(* Logix 5000 AddOnInstructionDefinition export Banner_LM_Param_v4; software revision 33.00; part 2 of 2 *)
(* tags used below, declared in another part *)
   LM : Banner_LM_v4;
   Port_Data : Banner_IOL_Port_v4;
   Port : INT;
   Local_Control : DINT;
   Command_Being_Processed : BOOL;
   Update_Archive : BOOL;
   Index_Write_Inprocess : INT;
   Index_Write_Control : INT;
   Inprocess_Index : DINT;
(* Banner_LM_Param_v4, continued *)

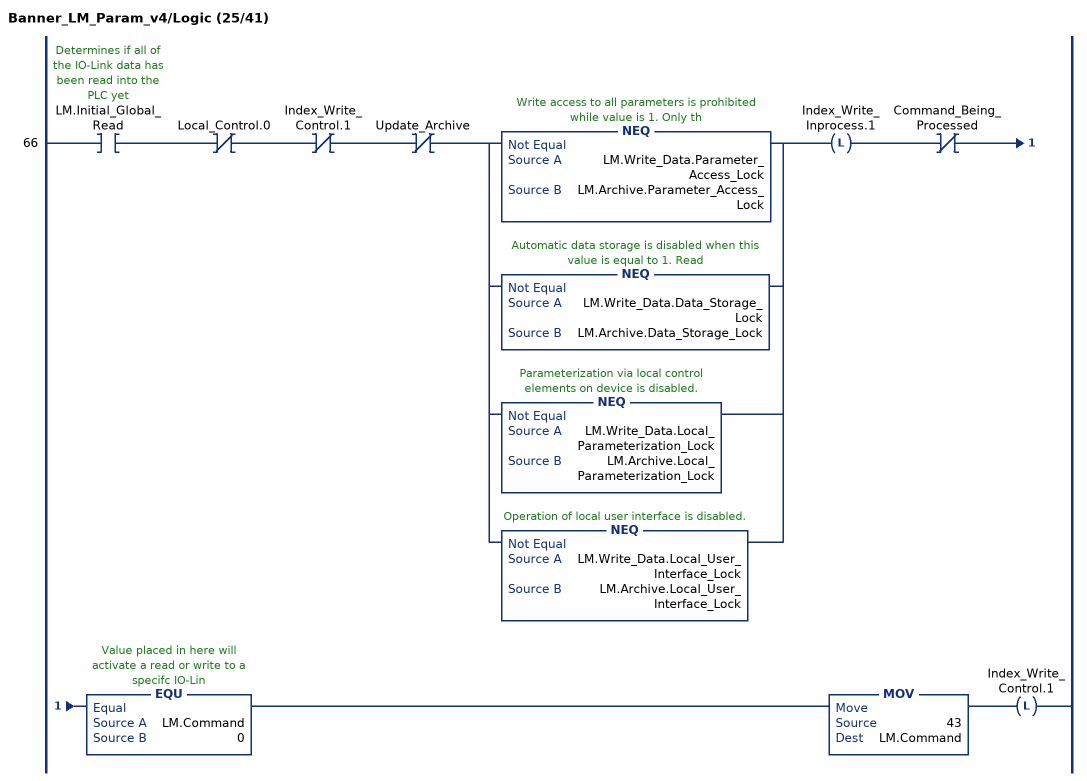
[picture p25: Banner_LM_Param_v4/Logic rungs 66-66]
   66: XIC(LM.Initial_Global_Read)XIO(Local_Control.0)XIO(Index_Write_Control.1)XIO(Update_Archive)[NEQ(LM.Write_Data.Parameter_Access_Lock,LM.Archive.Parameter_Access_Lock) ,NEQ(LM.Write_Data.Data_Storage_Lock,LM.Archive.Data_Storage_Lock) ,NEQ(LM.Write_Data.Local_Parameterization_Lock,LM.Archive.Local_Parameterization_Lock) ,NEQ(LM.Write_Data.Local_User_Interface_Lock,LM.Archive.Local_User_Interface_Lock) ]OTL(Index_Write_Inprocess.1)XIO(Command_Being_Processed)EQU(LM.Command,0)MOV(43,LM.Command)OTL(Index_Write_Control.1);
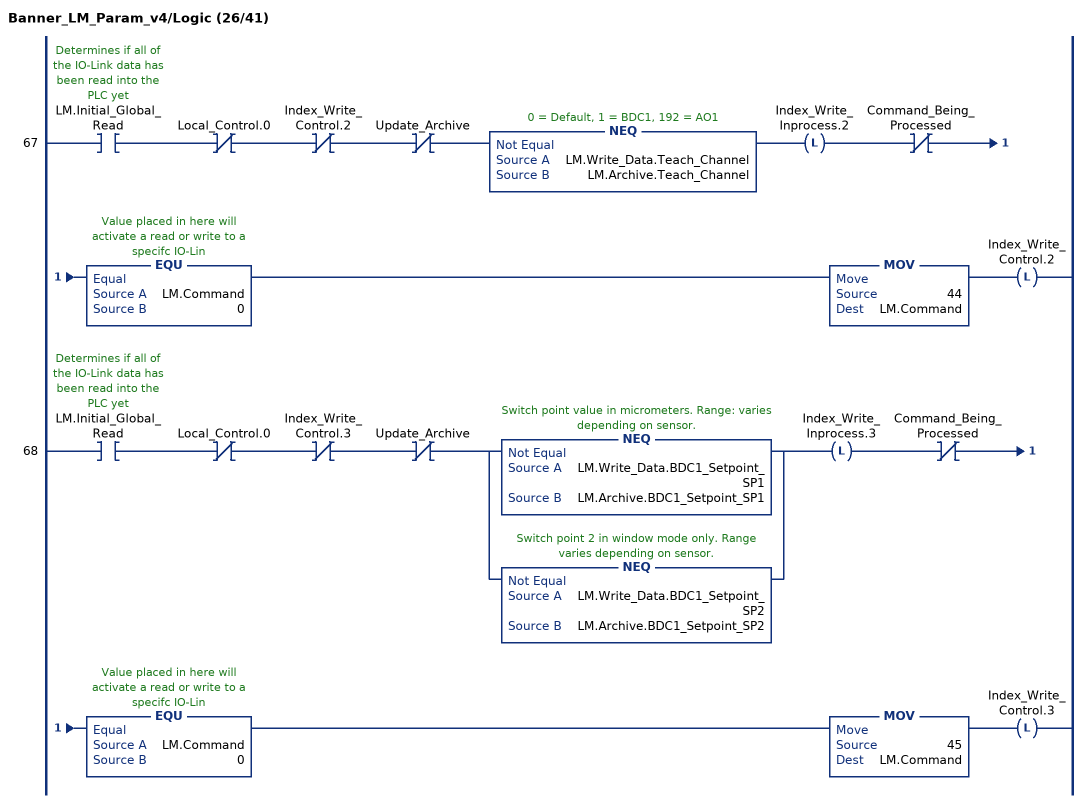
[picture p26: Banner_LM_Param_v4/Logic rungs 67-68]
   67: XIC(LM.Initial_Global_Read)XIO(Local_Control.0)XIO(Index_Write_Control.2)XIO(Update_Archive)NEQ(LM.Write_Data.Teach_Channel,LM.Archive.Teach_Channel)OTL(Index_Write_Inprocess.2)XIO(Command_Being_Processed)EQU(LM.Command,0)MOV(44,LM.Command)OTL(Index_Write_Control.2);
   68: XIC(LM.Initial_Global_Read)XIO(Local_Control.0)XIO(Index_Write_Control.3)XIO(Update_Archive)[NEQ(LM.Write_Data.BDC1_Setpoint_SP1,LM.Archive.BDC1_Setpoint_SP1) ,NEQ(LM.Write_Data.BDC1_Setpoint_SP2,LM.Archive.BDC1_Setpoint_SP2) ]OTL(Index_Write_Inprocess.3)XIO(Command_Being_Processed)EQU(LM.Command,0)MOV(45,LM.Command)OTL(Index_Write_Control.3);
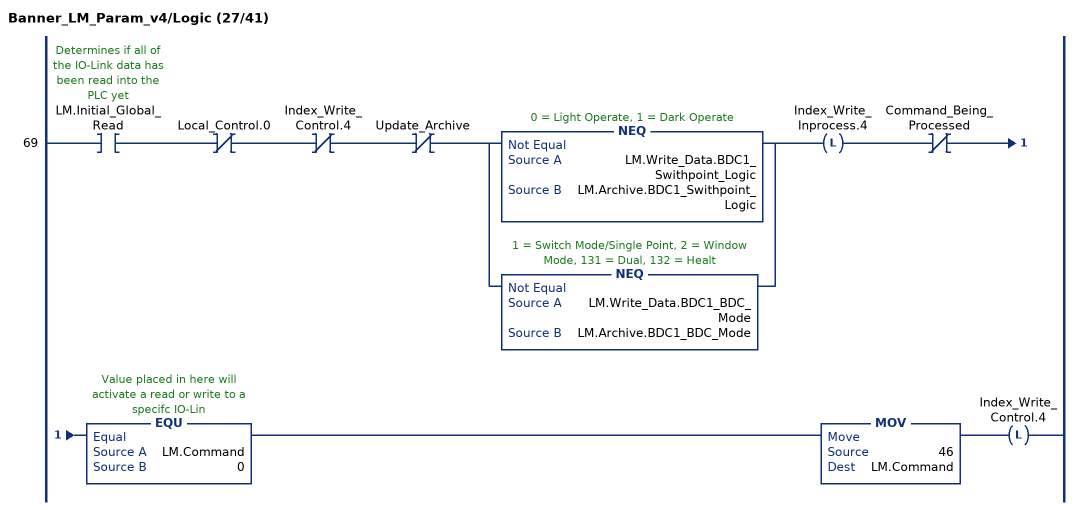
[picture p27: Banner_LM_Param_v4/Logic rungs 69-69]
   69: XIC(LM.Initial_Global_Read)XIO(Local_Control.0)XIO(Index_Write_Control.4)XIO(Update_Archive)[NEQ(LM.Write_Data.BDC1_Swithpoint_Logic,LM.Archive.BDC1_Swithpoint_Logic) ,NEQ(LM.Write_Data.BDC1_BDC_Mode,LM.Archive.BDC1_BDC_Mode) ]OTL(Index_Write_Inprocess.4)XIO(Command_Being_Processed)EQU(LM.Command,0)MOV(46,LM.Command)OTL(Index_Write_Control.4);
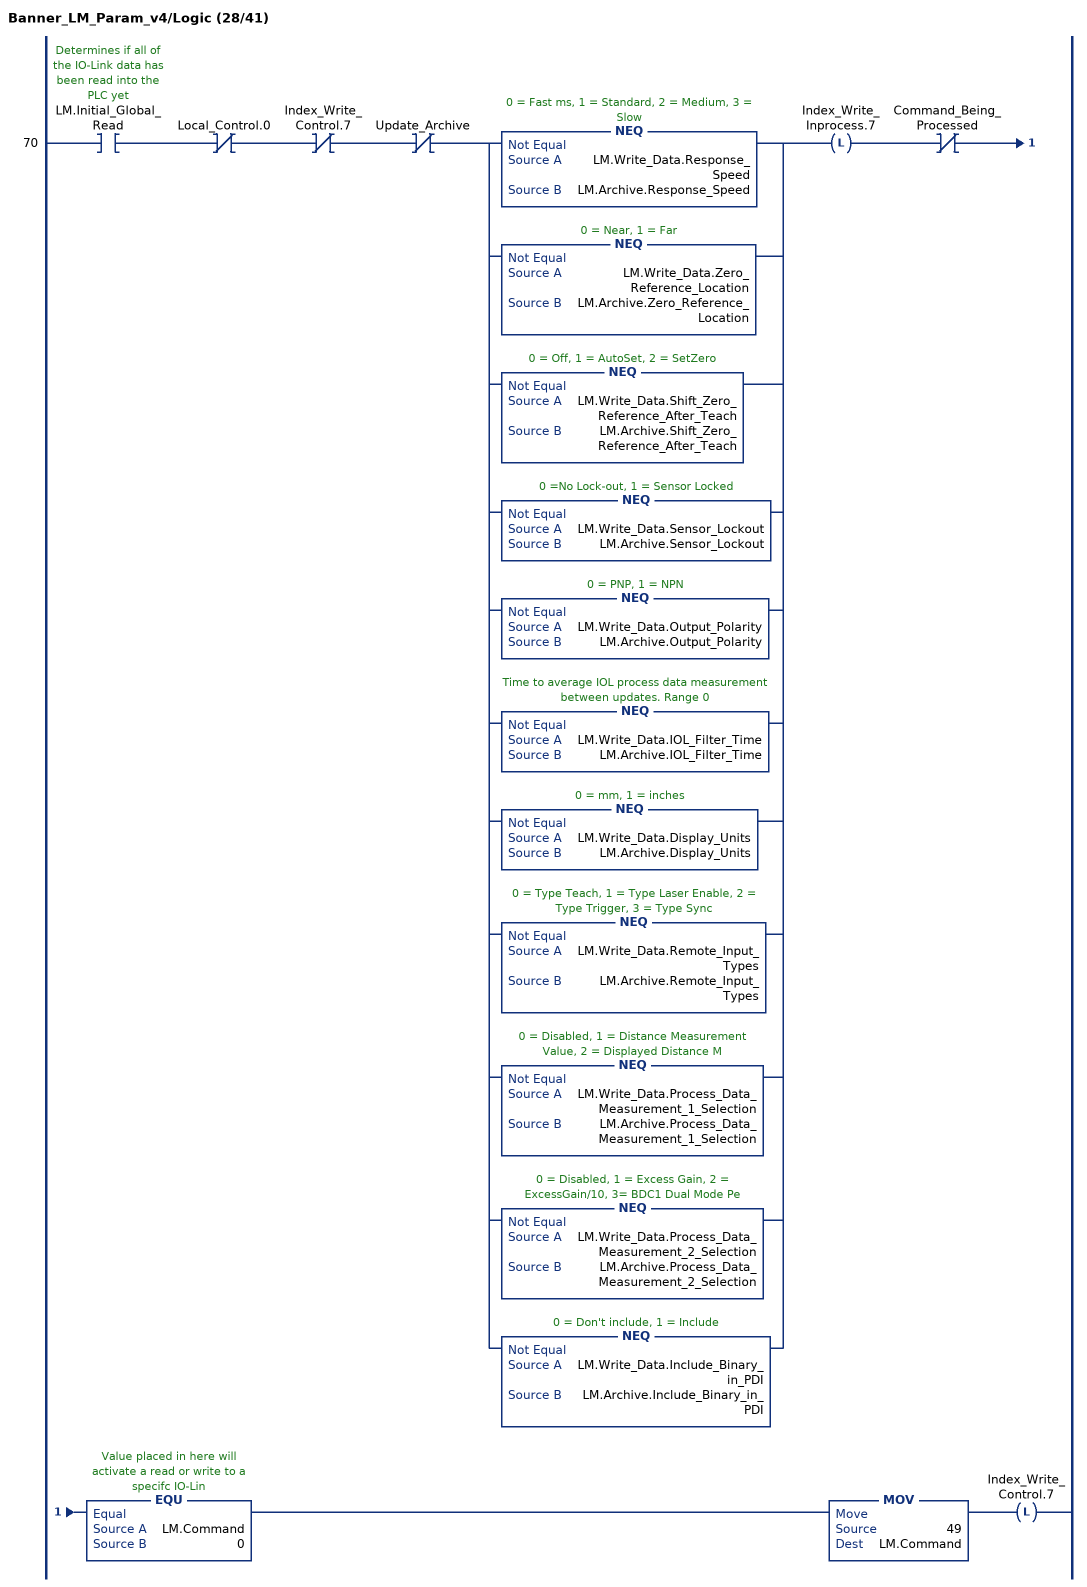
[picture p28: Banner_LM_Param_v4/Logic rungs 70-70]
   70: XIC(LM.Initial_Global_Read)XIO(Local_Control.0)XIO(Index_Write_Control.7)XIO(Update_Archive)[NEQ(LM.Write_Data.Response_Speed,LM.Archive.Response_Speed) ,NEQ(LM.Write_Data.Zero_Reference_Location,LM.Archive.Zero_Reference_Location) ,NEQ(LM.Write_Data.Shift_Zero_Reference_After_Teach,LM.Archive.Shift_Zero_Reference_After_Teach) ,NEQ(LM.Write_Data.Sensor_Lockout,LM.Archive.Sensor_Lockout) ,NEQ(LM.Write_Data.Output_Polarity,LM.Archive.Output_Polarity) ,NEQ(LM.Write_Data.IOL_Filter_Time,LM.Archive.IOL_Filter_Time) ,NEQ(LM.Write_Data.Display_Units,LM.Archive.Display_Units) ,NEQ(LM.Write_Data.Remote_Input_Types,LM.Archive.Remote_Input_Types) ,NEQ(LM.Write_Data.Process_Data_Measurement_1_Selection,LM.Archive.Process_Data_Measurement_1_Selection) ,NEQ(LM.Write_Data.Process_Data_Measurement_2_Selection,LM.Archive.Process_Data_Measurement_2_Selection) ,NEQ(LM.Write_Data.Include_Binary_in_PDI,LM.Archive.Include_Binary_in_PDI) ]OTL(Index_Write_Inprocess.7)XIO(Command_Being_Processed)EQU(LM.Command,0)MOV(49,LM.Command)OTL(Index_Write_Control.7);
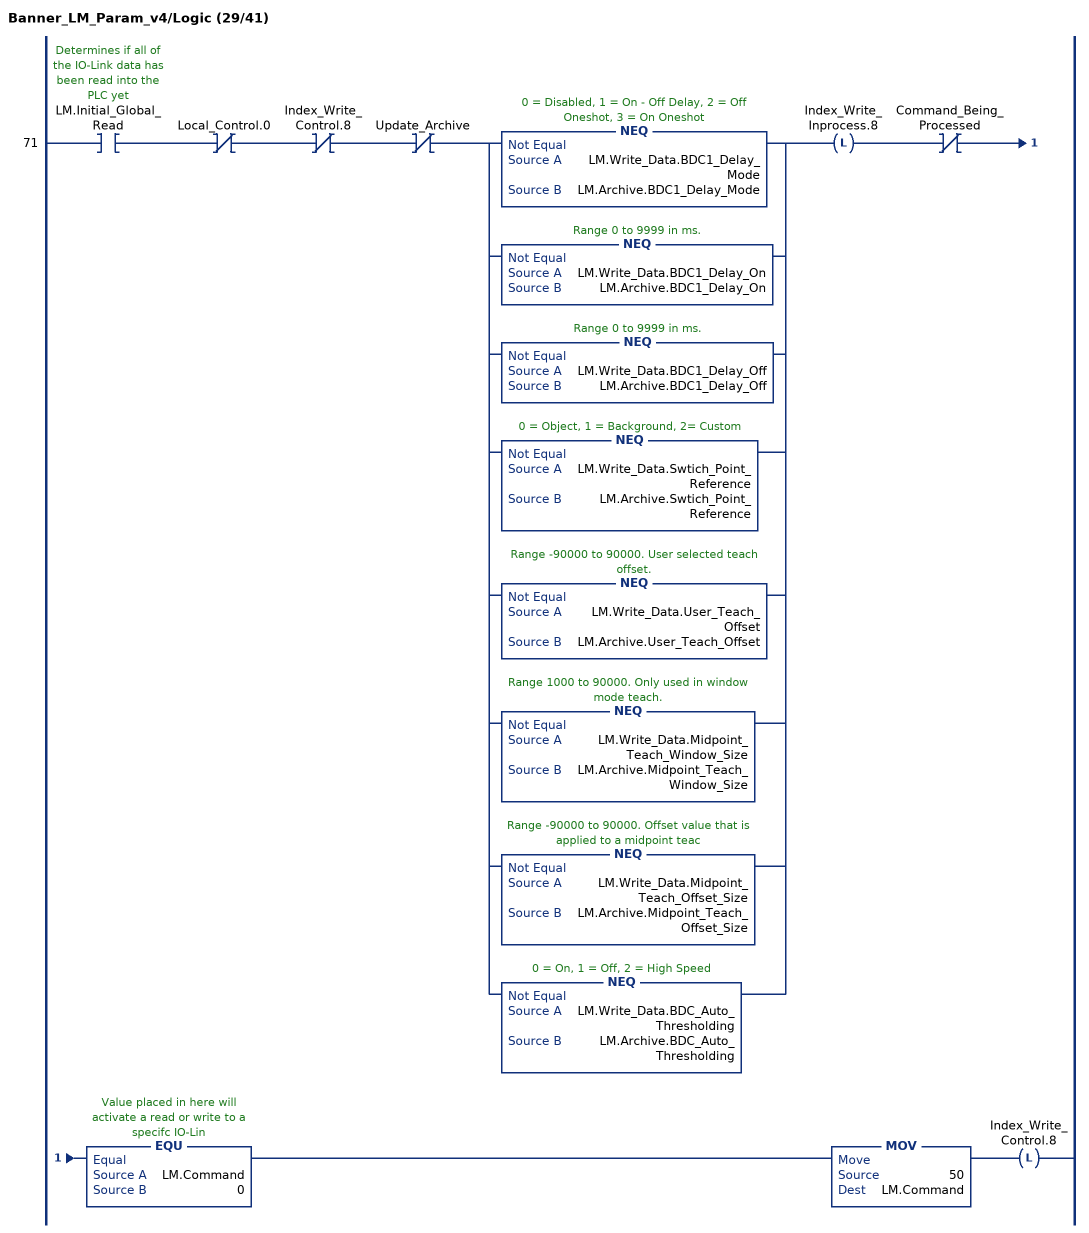
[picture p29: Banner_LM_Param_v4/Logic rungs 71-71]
   71: XIC(LM.Initial_Global_Read)XIO(Local_Control.0)XIO(Index_Write_Control.8)XIO(Update_Archive)[NEQ(LM.Write_Data.BDC1_Delay_Mode,LM.Archive.BDC1_Delay_Mode) ,NEQ(LM.Write_Data.BDC1_Delay_On,LM.Archive.BDC1_Delay_On) ,NEQ(LM.Write_Data.BDC1_Delay_Off,LM.Archive.BDC1_Delay_Off) ,NEQ(LM.Write_Data.Swtich_Point_Reference,LM.Archive.Swtich_Point_Reference) ,NEQ(LM.Write_Data.User_Teach_Offset,LM.Archive.User_Teach_Offset) ,NEQ(LM.Write_Data.Midpoint_Teach_Window_Size,LM.Archive.Midpoint_Teach_Window_Size) ,NEQ(LM.Write_Data.Midpoint_Teach_Offset_Size,LM.Archive.Midpoint_Teach_Offset_Size) ,NEQ(LM.Write_Data.BDC_Auto_Thresholding,LM.Archive.BDC_Auto_Thresholding) ]OTL(Index_Write_Inprocess.8)XIO(Command_Being_Processed)EQU(LM.Command,0)MOV(50,LM.Command)OTL(Index_Write_Control.8);
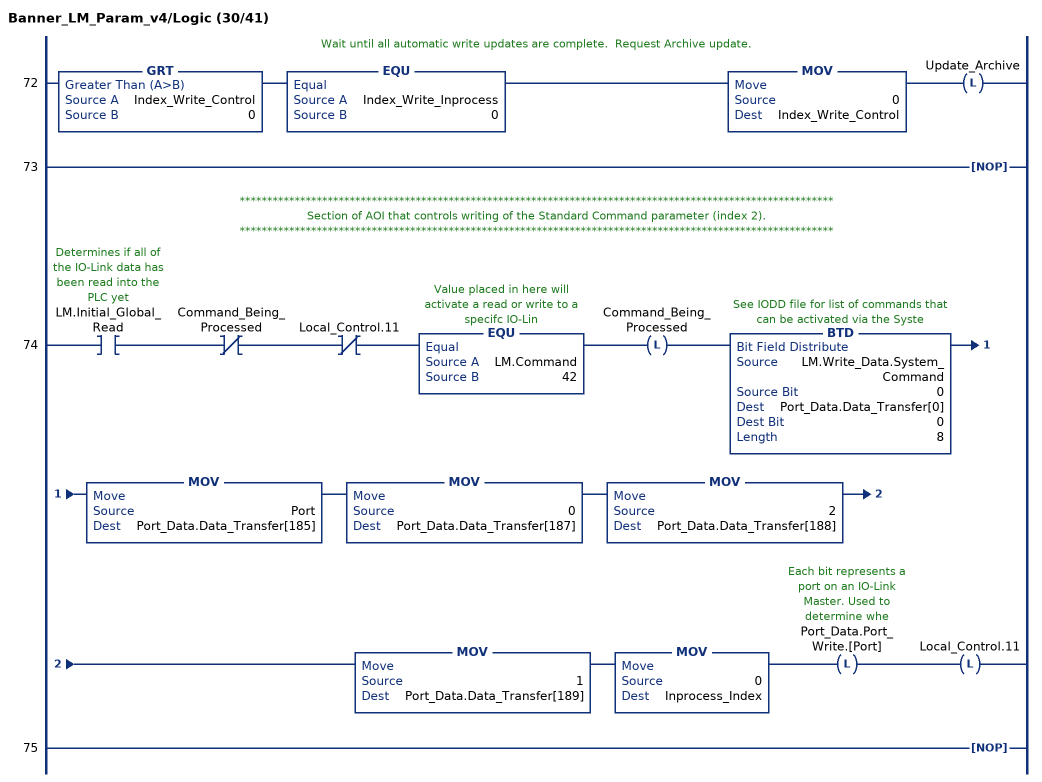
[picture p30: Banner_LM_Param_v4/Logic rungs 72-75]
   // Wait until all automatic write updates are complete.  Request Archive update.
   72: GRT(Index_Write_Control,0)EQU(Index_Write_Inprocess,0)MOV(0,Index_Write_Control)OTL(Update_Archive);
   73: NOP();
   // ************************************************************************************************************
   // Section of AOI that controls writing of the Standard Command parameter (index 2).
   // ************************************************************************************************************
   74: XIC(LM.Initial_Global_Read)XIO(Command_Being_Processed)XIO(Local_Control.11)EQU(LM.Command,42)OTL(Command_Being_Processed)BTD(LM.Write_Data.System_Command,0,Port_Data.Data_Transfer[0],0,8)MOV(Port,Port_Data.Data_Transfer[185])MOV(0,Port_Data.Data_Transfer[187])MOV(2,Port_Data.Data_Transfer[188])MOV(1,Port_Data.Data_Transfer[189])MOV(0,Inprocess_Index)OTL(Port_Data.Port_Write.[Port])OTL(Local_Control.11);
   75: NOP();
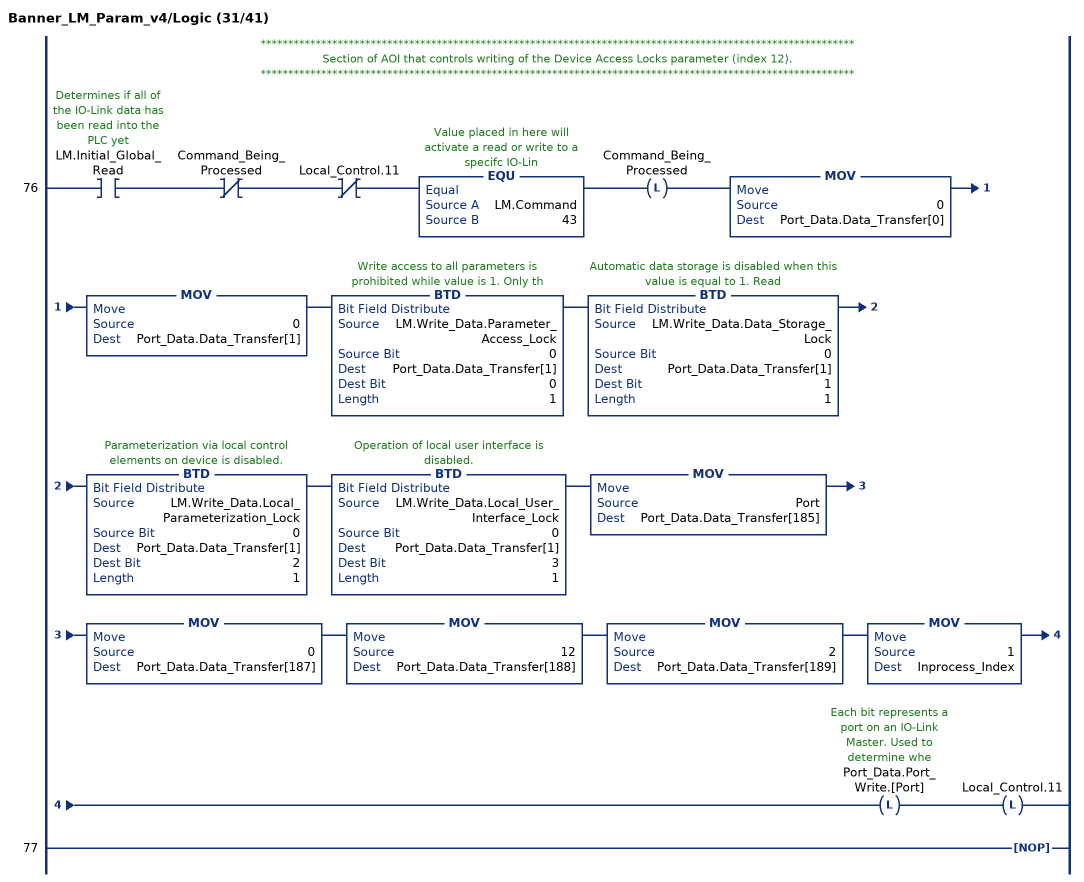
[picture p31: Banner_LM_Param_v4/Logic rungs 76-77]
   // ************************************************************************************************************
   // Section of AOI that controls writing of the Device Access Locks parameter (index 12).
   // ************************************************************************************************************
   76: XIC(LM.Initial_Global_Read)XIO(Command_Being_Processed)XIO(Local_Control.11)EQU(LM.Command,43)OTL(Command_Being_Processed)MOV(0,Port_Data.Data_Transfer[0])MOV(0,Port_Data.Data_Transfer[1])BTD(LM.Write_Data.Parameter_Access_Lock,0,Port_Data.Data_Transfer[1],0,1)BTD(LM.Write_Data.Data_Storage_Lock,0,Port_Data.Data_Transfer[1],1,1)BTD(LM.Write_Data.Local_Parameterization_Lock,0,Port_Data.Data_Transfer[1],2,1)BTD(LM.Write_Data.Local_User_Interface_Lock,0,Port_Data.Data_Transfer[1],3,1)MOV(Port,Port_Data.Data_Transfer[185])MOV(0,Port_Data.Data_Transfer[187])MOV(12,Port_Data.Data_Transfer[188])MOV(2,Port_Data.Data_Transfer[189])MOV(1,Inprocess_Index)OTL(Port_Data.Port_Write.[Port])OTL(Local_Control.11);
   77: NOP();
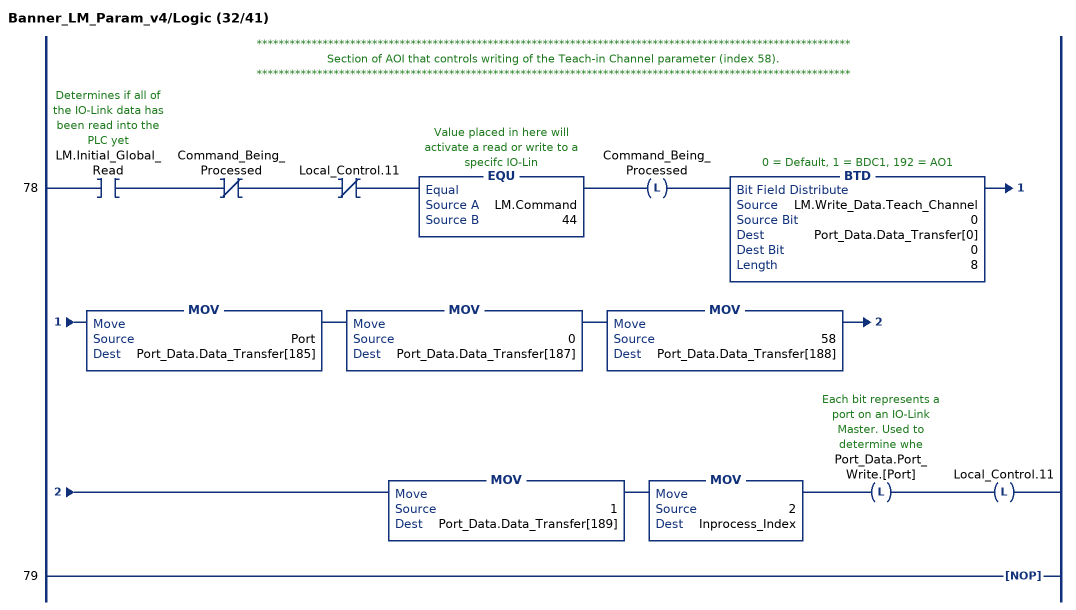
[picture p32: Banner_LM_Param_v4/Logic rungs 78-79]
   // ************************************************************************************************************
   // Section of AOI that controls writing of the Teach-in Channel parameter (index 58).
   // ************************************************************************************************************
   78: XIC(LM.Initial_Global_Read)XIO(Command_Being_Processed)XIO(Local_Control.11)EQU(LM.Command,44)OTL(Command_Being_Processed)BTD(LM.Write_Data.Teach_Channel,0,Port_Data.Data_Transfer[0],0,8)MOV(Port,Port_Data.Data_Transfer[185])MOV(0,Port_Data.Data_Transfer[187])MOV(58,Port_Data.Data_Transfer[188])MOV(1,Port_Data.Data_Transfer[189])MOV(2,Inprocess_Index)OTL(Port_Data.Port_Write.[Port])OTL(Local_Control.11);
   79: NOP();
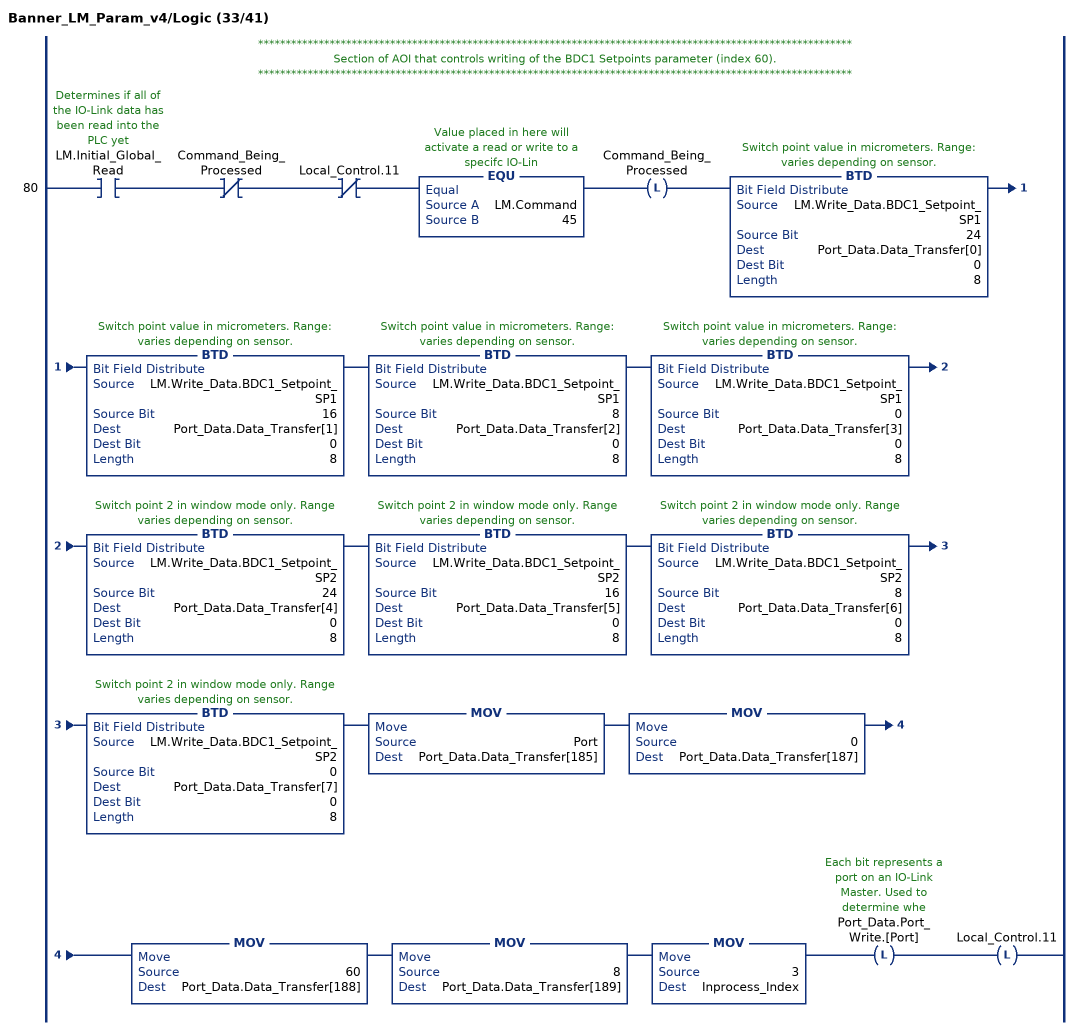
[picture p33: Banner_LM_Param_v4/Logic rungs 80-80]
   // ************************************************************************************************************
   // Section of AOI that controls writing of the BDC1 Setpoints parameter (index 60).
   // ************************************************************************************************************
   80: XIC(LM.Initial_Global_Read)XIO(Command_Being_Processed)XIO(Local_Control.11)EQU(LM.Command,45)OTL(Command_Being_Processed)BTD(LM.Write_Data.BDC1_Setpoint_SP1,24,Port_Data.Data_Transfer[0],0,8)BTD(LM.Write_Data.BDC1_Setpoint_SP1,16,Port_Data.Data_Transfer[1],0,8)BTD(LM.Write_Data.BDC1_Setpoint_SP1,8,Port_Data.Data_Transfer[2],0,8)BTD(LM.Write_Data.BDC1_Setpoint_SP1,0,Port_Data.Data_Transfer[3],0,8)BTD(LM.Write_Data.BDC1_Setpoint_SP2,24,Port_Data.Data_Transfer[4],0,8)BTD(LM.Write_Data.BDC1_Setpoint_SP2,16,Port_Data.Data_Transfer[5],0,8)BTD(LM.Write_Data.BDC1_Setpoint_SP2,8,Port_Data.Data_Transfer[6],0,8)BTD(LM.Write_Data.BDC1_Setpoint_SP2,0,Port_Data.Data_Transfer[7],0,8)MOV(Port,Port_Data.Data_Transfer[185])MOV(0,Port_Data.Data_Transfer[187])MOV(60,Port_Data.Data_Transfer[188])MOV(8,Port_Data.Data_Transfer[189])MOV(3,Inprocess_Index)OTL(Port_Data.Port_Write.[Port])OTL(Local_Control.11);
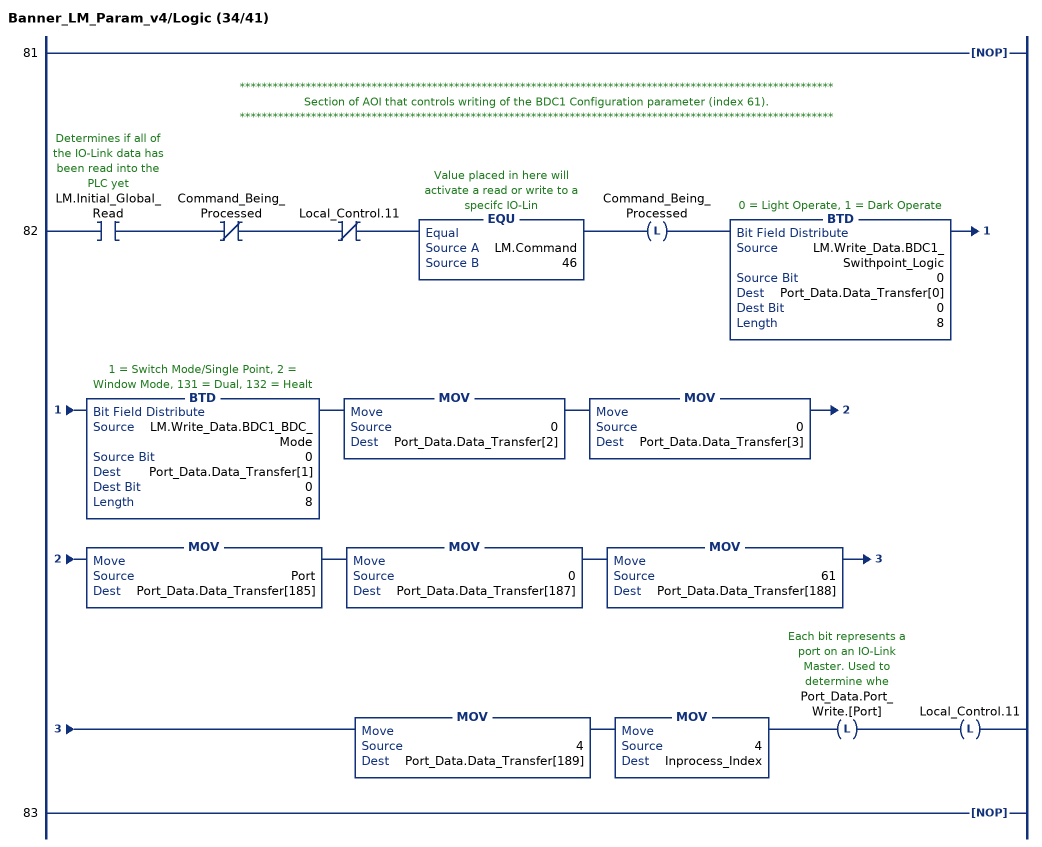
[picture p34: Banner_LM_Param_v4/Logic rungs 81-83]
   81: NOP();
   // ************************************************************************************************************
   // Section of AOI that controls writing of the BDC1 Configuration parameter (index 61).
   // ************************************************************************************************************
   82: XIC(LM.Initial_Global_Read)XIO(Command_Being_Processed)XIO(Local_Control.11)EQU(LM.Command,46)OTL(Command_Being_Processed)BTD(LM.Write_Data.BDC1_Swithpoint_Logic,0,Port_Data.Data_Transfer[0],0,8)BTD(LM.Write_Data.BDC1_BDC_Mode,0,Port_Data.Data_Transfer[1],0,8)MOV(0,Port_Data.Data_Transfer[2])MOV(0,Port_Data.Data_Transfer[3])MOV(Port,Port_Data.Data_Transfer[185])MOV(0,Port_Data.Data_Transfer[187])MOV(61,Port_Data.Data_Transfer[188])MOV(4,Port_Data.Data_Transfer[189])MOV(4,Inprocess_Index)OTL(Port_Data.Port_Write.[Port])OTL(Local_Control.11);
   83: NOP();
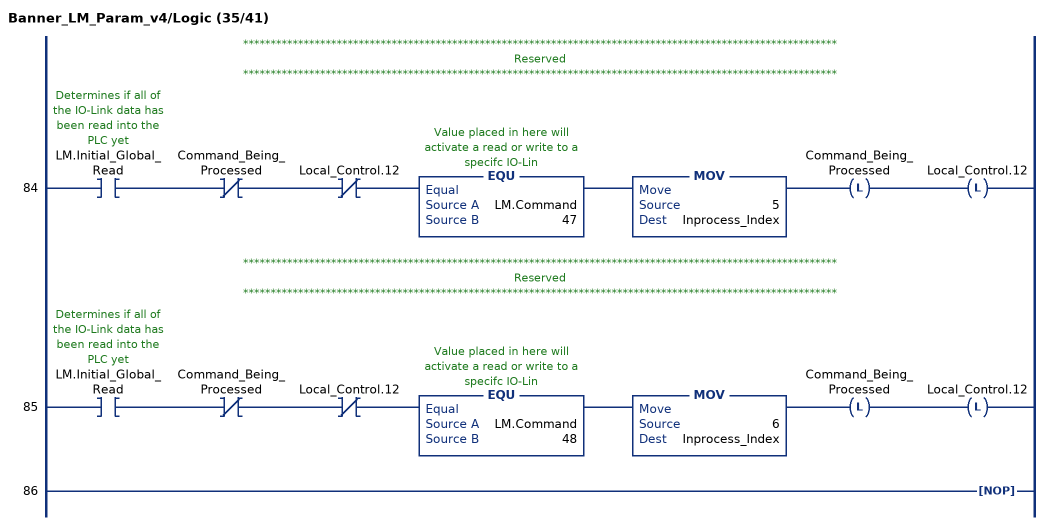
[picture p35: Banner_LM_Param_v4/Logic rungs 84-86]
   // ************************************************************************************************************
   // Reserved
   // ************************************************************************************************************
   84: XIC(LM.Initial_Global_Read)XIO(Command_Being_Processed)XIO(Local_Control.12)EQU(LM.Command,47)MOV(5,Inprocess_Index)OTL(Command_Being_Processed)OTL(Local_Control.12);
   // ************************************************************************************************************
   // Reserved
   // ************************************************************************************************************
   85: XIC(LM.Initial_Global_Read)XIO(Command_Being_Processed)XIO(Local_Control.12)EQU(LM.Command,48)MOV(6,Inprocess_Index)OTL(Command_Being_Processed)OTL(Local_Control.12);
   86: NOP();
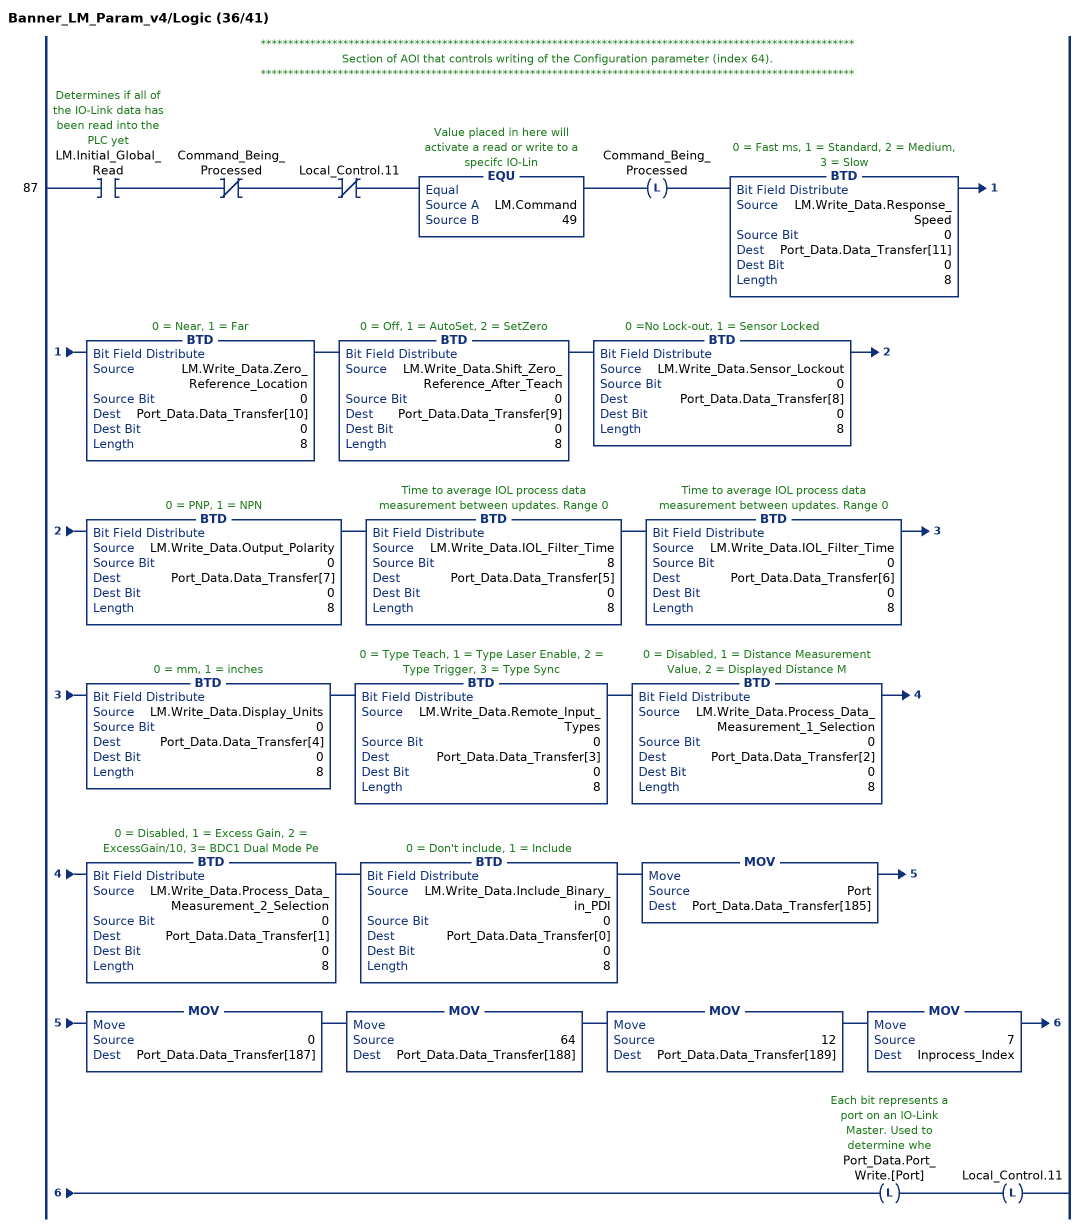
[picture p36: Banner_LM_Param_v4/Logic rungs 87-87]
   // ************************************************************************************************************
   // Section of AOI that controls writing of the Configuration parameter (index 64).
   // ************************************************************************************************************
   87: XIC(LM.Initial_Global_Read)XIO(Command_Being_Processed)XIO(Local_Control.11)EQU(LM.Command,49)OTL(Command_Being_Processed)BTD(LM.Write_Data.Response_Speed,0,Port_Data.Data_Transfer[11],0,8)BTD(LM.Write_Data.Zero_Reference_Location,0,Port_Data.Data_Transfer[10],0,8)BTD(LM.Write_Data.Shift_Zero_Reference_After_Teach,0,Port_Data.Data_Transfer[9],0,8)BTD(LM.Write_Data.Sensor_Lockout,0,Port_Data.Data_Transfer[8],0,8)BTD(LM.Write_Data.Output_Polarity,0,Port_Data.Data_Transfer[7],0,8)BTD(LM.Write_Data.IOL_Filter_Time,8,Port_Data.Data_Transfer[5],0,8)BTD(LM.Write_Data.IOL_Filter_Time,0,Port_Data.Data_Transfer[6],0,8)BTD(LM.Write_Data.Display_Units,0,Port_Data.Data_Transfer[4],0,8)BTD(LM.Write_Data.Remote_Input_Types,0,Port_Data.Data_Transfer[3],0,8)BTD(LM.Write_Data.Process_Data_Measurement_1_Selection,0,Port_Data.Data_Transfer[2],0,8)BTD(LM.Write_Data.Process_Data_Measurement_2_Selection,0,Port_Data.Data_Transfer[1],0,8)BTD(LM.Write_Data.Include_Binary_in_PDI,0,Port_Data.Data_Transfer[0],0,8)MOV(Port,Port_Data.Data_Transfer[185])MOV(0,Port_Data.Data_Transfer[187])MOV(64,Port_Data.Data_Transfer[188])MOV(12,Port_Data.Data_Transfer[189])MOV(7,Inprocess_Index)OTL(Port_Data.Port_Write.[Port])OTL(Local_Control.11);
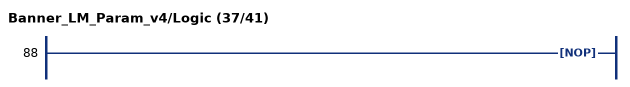
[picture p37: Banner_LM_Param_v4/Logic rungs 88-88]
   88: NOP();
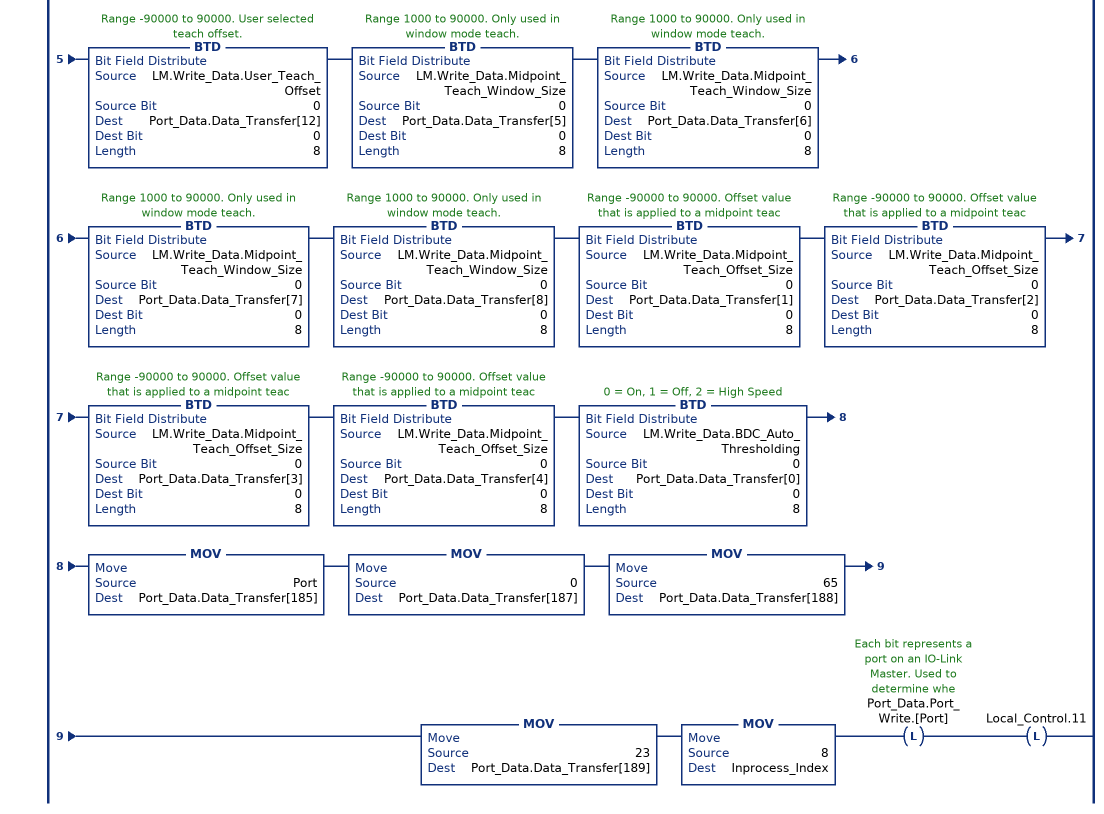
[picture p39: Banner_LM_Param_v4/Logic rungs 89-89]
   // ************************************************************************************************************
   // Section of AOI that controls writing of the BDC1 Vendor Specific Configuration parameter (index 65).
   // ************************************************************************************************************
   89: XIC(LM.Initial_Global_Read)XIO(Command_Being_Processed)XIO(Local_Control.11)EQU(LM.Command,50)OTL(Command_Being_Processed)BTD(LM.Write_Data.BDC1_Delay_Mode,0,Port_Data.Data_Transfer[22],0,8)BTD(LM.Write_Data.BDC1_Delay_On,0,Port_Data.Data_Transfer[18],0,8)BTD(LM.Write_Data.BDC1_Delay_On,0,Port_Data.Data_Transfer[19],0,8)BTD(LM.Write_Data.BDC1_Delay_On,0,Port_Data.Data_Transfer[20],0,8)BTD(LM.Write_Data.BDC1_Delay_On,0,Port_Data.Data_Transfer[21],0,8)BTD(LM.Write_Data.BDC1_Delay_Off,0,Port_Data.Data_Transfer[14],0,8)BTD(LM.Write_Data.BDC1_Delay_Off,0,Port_Data.Data_Transfer[15],0,8)BTD(LM.Write_Data.BDC1_Delay_Off,0,Port_Data.Data_Transfer[16],0,8)BTD(LM.Write_Data.BDC1_Delay_Off,0,Port_Data.Data_Transfer[17],0,8)BTD(LM.Write_Data.Swtich_Point_Reference,0,Port_Data.Data_Transfer[13],0,8)BTD(LM.Write_Data.User_Teach_Offset,0,Port_Data.Data_Transfer[9],0,8)BTD(LM.Write_Data.User_Teach_Offset,0,Port_Data.Data_Transfer[10],0,8)BTD(LM.Write_Data.User_Teach_Offset,0,Port_Data.Data_Transfer[11],0,8)BTD(LM.Write_Data.User_Teach_Offset,0,Port_Data.Data_Transfer[12],0,8)BTD(LM.Write_Data.Midpoint_Teach_Window_Size,0,Port_Data.Data_Transfer[5],0,8)BTD(LM.Write_Data.Midpoint_Teach_Window_Size,0,Port_Data.Data_Transfer[6],0,8)BTD(LM.Write_Data.Midpoint_Teach_Window_Size,0,Port_Data.Data_Transfer[7],0,8)BTD(LM.Write_Data.Midpoint_Teach_Window_Size,0,Port_Data.Data_Transfer[8],0,8)BTD(LM.Write_Data.Midpoint_Teach_Offset_Size,0,Port_Data.Data_Transfer[1],0,8)BTD(LM.Write_Data.Midpoint_Teach_Offset_Size,0,Port_Data.Data_Transfer[2],0,8)BTD(LM.Write_Data.Midpoint_Teach_Offset_Size,0,Port_Data.Data_Transfer[3],0,8)BTD(LM.Write_Data.Midpoint_Teach_Offset_Size,0,Port_Data.Data_Transfer[4],0,8)BTD(LM.Write_Data.BDC_Auto_Thresholding,0,Port_Data.Data_Transfer[0],0,8)MOV(Port,Port_Data.Data_Transfer[185])MOV(0,Port_Data.Data_Transfer[187])MOV(65,Port_Data.Data_Transfer[188])MOV(23,Port_Data.Data_Transfer[189])MOV(8,Inprocess_Index)OTL(Port_Data.Port_Write.[Port])OTL(Local_Control.11);
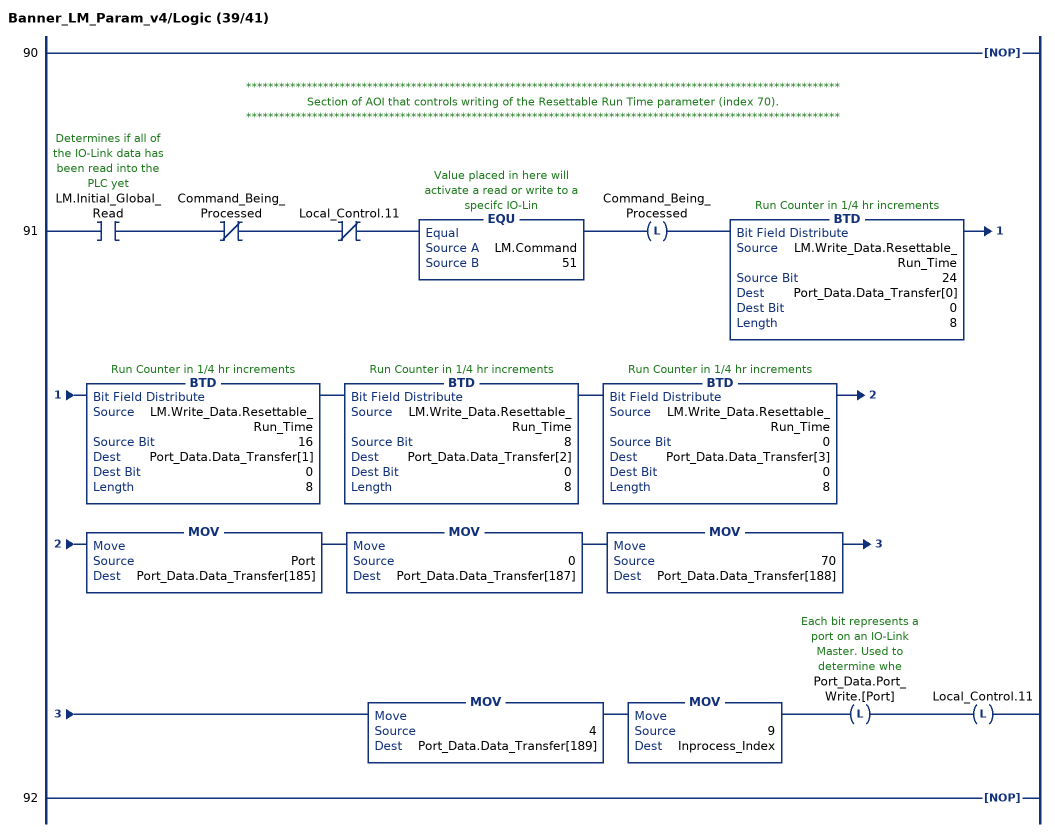
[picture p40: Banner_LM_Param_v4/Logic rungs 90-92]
   90: NOP();
   // ************************************************************************************************************
   // Section of AOI that controls writing of the Resettable Run Time parameter (index 70).
   // ************************************************************************************************************
   91: XIC(LM.Initial_Global_Read)XIO(Command_Being_Processed)XIO(Local_Control.11)EQU(LM.Command,51)OTL(Command_Being_Processed)BTD(LM.Write_Data.Resettable_Run_Time,24,Port_Data.Data_Transfer[0],0,8)BTD(LM.Write_Data.Resettable_Run_Time,16,Port_Data.Data_Transfer[1],0,8)BTD(LM.Write_Data.Resettable_Run_Time,8,Port_Data.Data_Transfer[2],0,8)BTD(LM.Write_Data.Resettable_Run_Time,0,Port_Data.Data_Transfer[3],0,8)MOV(Port,Port_Data.Data_Transfer[185])MOV(0,Port_Data.Data_Transfer[187])MOV(70,Port_Data.Data_Transfer[188])MOV(4,Port_Data.Data_Transfer[189])MOV(9,Inprocess_Index)OTL(Port_Data.Port_Write.[Port])OTL(Local_Control.11);
   92: NOP();
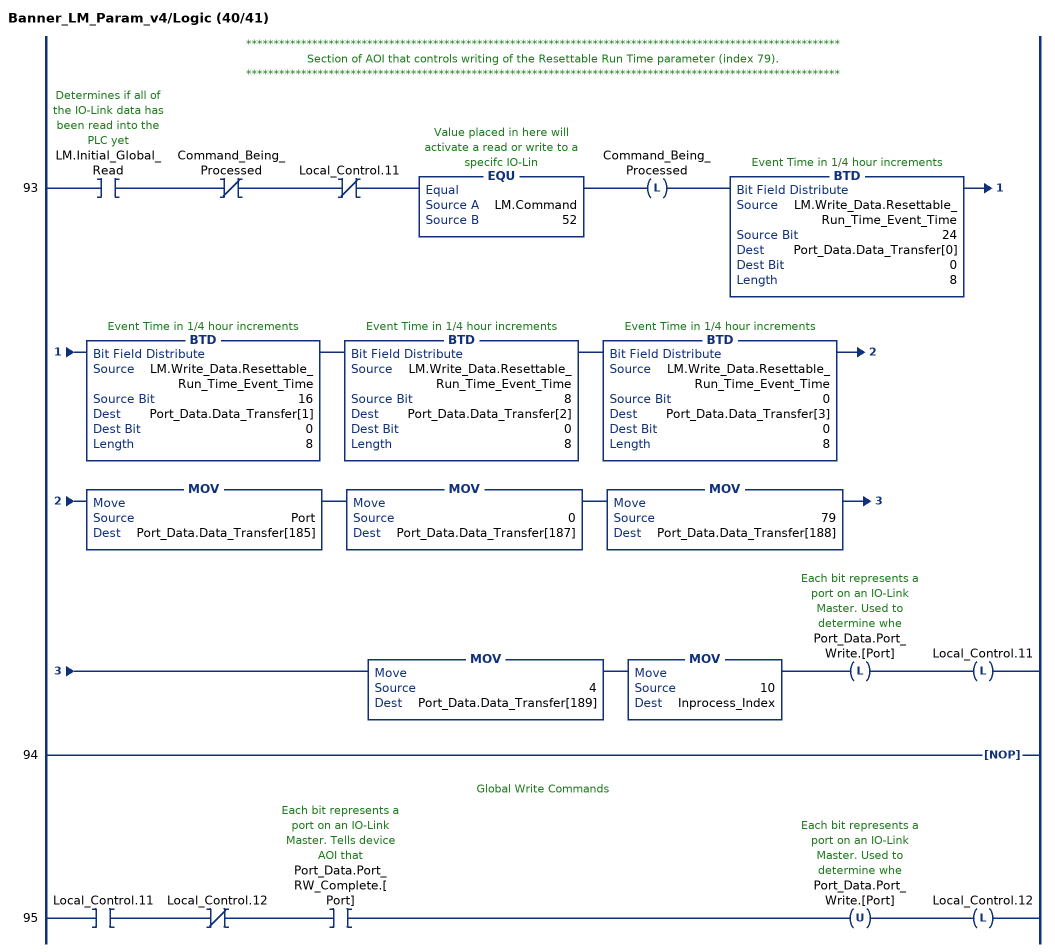
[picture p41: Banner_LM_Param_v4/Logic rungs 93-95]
   // ************************************************************************************************************
   // Section of AOI that controls writing of the Resettable Run Time parameter (index 79).
   // ************************************************************************************************************
   93: XIC(LM.Initial_Global_Read)XIO(Command_Being_Processed)XIO(Local_Control.11)EQU(LM.Command,52)OTL(Command_Being_Processed)BTD(LM.Write_Data.Resettable_Run_Time_Event_Time,24,Port_Data.Data_Transfer[0],0,8)BTD(LM.Write_Data.Resettable_Run_Time_Event_Time,16,Port_Data.Data_Transfer[1],0,8)BTD(LM.Write_Data.Resettable_Run_Time_Event_Time,8,Port_Data.Data_Transfer[2],0,8)BTD(LM.Write_Data.Resettable_Run_Time_Event_Time,0,Port_Data.Data_Transfer[3],0,8)MOV(Port,Port_Data.Data_Transfer[185])MOV(0,Port_Data.Data_Transfer[187])MOV(79,Port_Data.Data_Transfer[188])MOV(4,Port_Data.Data_Transfer[189])MOV(10,Inprocess_Index)OTL(Port_Data.Port_Write.[Port])OTL(Local_Control.11);
   94: NOP();
   // Global Write Commands
   95: XIC(Local_Control.11)XIO(Local_Control.12)XIC(Port_Data.Port_RW_Complete.[Port])OTU(Port_Data.Port_Write.[Port])OTL(Local_Control.12);
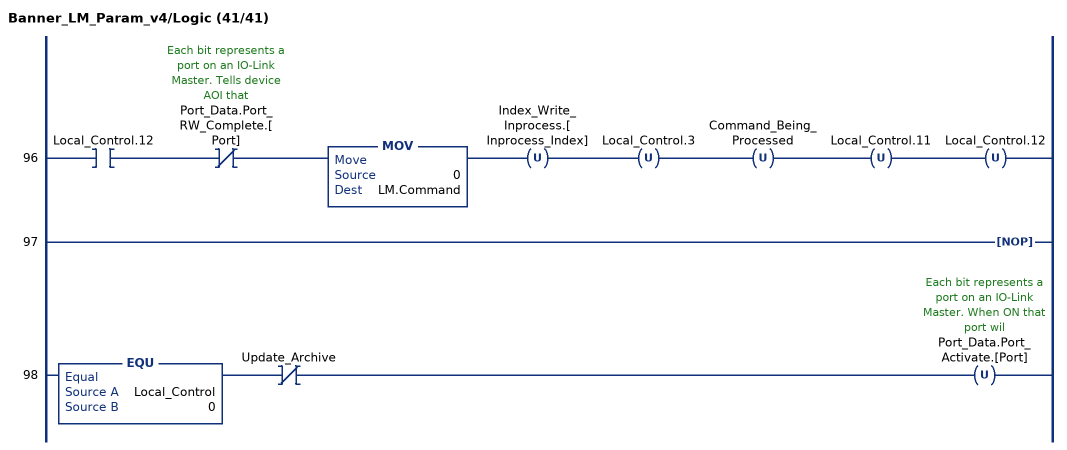
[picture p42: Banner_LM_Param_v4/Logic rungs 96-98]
   96: XIC(Local_Control.12)XIO(Port_Data.Port_RW_Complete.[Port])MOV(0,LM.Command)OTU(Index_Write_Inprocess.[Inprocess_Index])OTU(Local_Control.3)OTU(Command_Being_Processed)OTU(Local_Control.11)OTU(Local_Control.12);
   97: NOP();
   98: EQU(Local_Control,0)XIO(Update_Archive)OTU(Port_Data.Port_Activate.[Port]);
END_ROUTINE
END_ADD_ON_INSTRUCTION
